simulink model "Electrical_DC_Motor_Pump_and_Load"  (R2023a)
settings: Solver=VariableStepAuto  StartTime=0.0  StopTime=10.0  RelTol=1e-3
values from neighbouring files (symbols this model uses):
  K_q = 1    [Electrical_DC_Motor_Pump_and_Load_EQN.m]    (also in Electrical_DC_Motor_Pump_and_Load_SLX_m.m; Electrical_DC_Motor_and_Pump_EQN.m; Electrical_DC_Motor_and_Pump_SLX_m.m)
  K_t = 1    [Electrical_DC_Motor_Pump_and_Load_EQN.m]    (also in Electrical_DC_Motor_Pump_and_Load_SLX_m.m; Electrical_DC_Motor_and_Pump_EQN.m; Electrical_DC_Motor_and_Pump_SLX_m.m)
undefined symbols (not defined in the file or in its folder): eTr, rGi
libraries: fl_lib x14

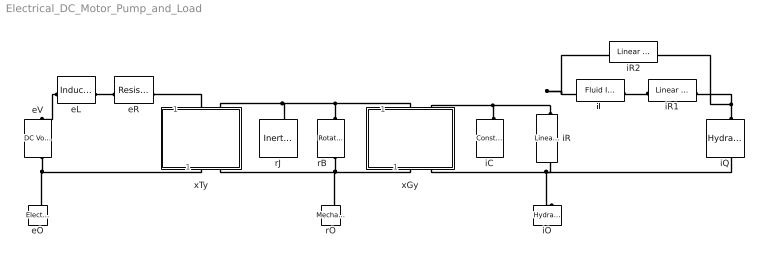
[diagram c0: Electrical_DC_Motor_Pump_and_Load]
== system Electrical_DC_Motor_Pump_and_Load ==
  eL : fl_lib/Electrical/Electrical Elements/Inductor  l=1e-6 H  r=0 Ohm  g=1e-9 1/Ohm  i_specify=off  i_priority=None  i=0 A  i_nominal_specify=off  i_nominal_unit=A  i_nominal_value=1  v_specify=off  v_priority=None  v=0 V  v_nominal_specify=off  v_nominal_unit=V  v_nominal_value=1  i_L_specify=off  i_L_priority=High  i_L=0 A  i_L_nominal_specify=off  i_L_nominal_unit=A  i_L_nominal_value=1
  eO : fl_lib/Electrical/Electrical Elements/Electrical Reference
  eR : fl_lib/Electrical/Electrical Elements/Resistor  R=1 Ohm  i_specify=off  i_priority=None  i=0 A  i_nominal_specify=off  i_nominal_unit=A  i_nominal_value=1  v_specify=off  v_priority=None  v=0 V  v_nominal_specify=off  v_nominal_unit=V  v_nominal_value=1
  eV : fl_lib/Electrical/Electrical Sources/DC Voltage Source  v0=1 V
  iC : fl_lib/Hydraulic/Hydraulic Elements/Constant Volume Hydraulic Chamber  ch_sp=foundation.enum.chamberGeometry.volume  wall_type=foundation.enum.chamber_spec.rigid  ch_volume=1e-4 m^3  d_in=1e-2 m  length=1 m  pr_r_coef=1.2e-12 m/Pa  time_const=0.01 s  k_sh=1.4  pressure_specify=off  pressure_priority=High  pressure=0 Pa  pressure_nominal_specify=off  pressure_nominal_unit=Pa  pressure_nominal_value=1  diameter_incr_specify=off  diameter_incr_priority=High  diameter_incr=0 m  diameter_incr_nominal_specify=off  diameter_incr_nominal_unit=m  diameter_incr_nominal_value=1  flow_rate_specify=off  flow_rate_priority=None  flow_rate=1e-3 m^3/s  flow_rate_nominal_specify=off  flow_rate_nominal_unit=m^3/s  flow_rate_nominal_value=1
  iL : fl_lib/Hydraulic/Hydraulic Elements/Fluid Inertia  area=0.8e-4 m^2  length=1 m  q_specify=off  q_priority=High  q=1e-3 m^3/s  q_nominal_specify=off  q_nominal_unit=m^3/s  q_nominal_value=1  p_specify=off  p_priority=None  p=0 Pa  p_nominal_specify=off  p_nominal_unit=Pa  p_nominal_value=1
  iO : fl_lib/Hydraulic/Hydraulic Elements/Hydraulic Reference
  iQ : fl_lib/Hydraulic/Hydraulic Sources/Hydraulic Constant Flow Rate Source  commanded_flow_rate=0.001 m^3/s
  iR : fl_lib/Hydraulic/Hydraulic Elements/Linear Hydraulic Resistance  resistance=10e9 Pa*s/m^3  q_specify=off  q_priority=None  q=1e-3 m^3/s  q_nominal_specify=off  q_nominal_unit=m^3/s  q_nominal_value=1  p_specify=off  p_priority=None  p=0 Pa  p_nominal_specify=off  p_nominal_unit=Pa  p_nominal_value=1
  iR1 : fl_lib/Hydraulic/Hydraulic Elements/Linear Hydraulic Resistance  resistance=10e9 Pa*s/m^3  q_specify=off  q_priority=None  q=1e-3 m^3/s  q_nominal_specify=off  q_nominal_unit=m^3/s  q_nominal_value=1  p_specify=off  p_priority=None  p=0 Pa  p_nominal_specify=off  p_nominal_unit=Pa  p_nominal_value=1
  iR2 : fl_lib/Hydraulic/Hydraulic Elements/Linear Hydraulic Resistance  resistance=10e9 Pa*s/m^3  q_specify=off  q_priority=None  q=1e-3 m^3/s  q_nominal_specify=off  q_nominal_unit=m^3/s  q_nominal_value=1  p_specify=off  p_priority=None  p=0 Pa  p_nominal_specify=off  p_nominal_unit=Pa  p_nominal_value=1
  rB : fl_lib/Mechanical/Rotational Elements/Rotational Damper  D=0.001 N*m*s/rad  w_specify=off  w_priority=None  w=0 rad/s  w_nominal_specify=off  w_nominal_unit=rad/s  w_nominal_value=1  t_specify=off  t_priority=None  t=0 N*m  t_nominal_specify=off  t_nominal_unit=N*m  t_nominal_value=1
  rJ : fl_lib/Mechanical/Rotational Elements/Inertia  inertia=0.01 kg*m^2  num_ports=foundation.enum.numPorts2.one  w_specify=off  w_priority=High  w=0 rad/s  w_nominal_specify=off  w_nominal_unit=rad/s  w_nominal_value=1  t_specify=off  t_priority=None  t=0 N*m  t_nominal_specify=off  t_nominal_unit=N*m  t_nominal_value=1
  rO : fl_lib/Mechanical/Rotational Elements/Mechanical Rotational Reference
  xGy : Subsystem  mask{Gyrator_type=rGi, G_type=F2=K*E1, xGy=K_q}
      mask prompts: Gyrator_type "Type of Gytator"; G_type "Type of relation"; xGy "Name of parameter K"
  xTy : Subsystem  mask{Transformer_type=eTr, T_type=F2=K*F1, xTy=K_t}
      mask prompts: Transformer_type "Type of Transformer"; T_type "Type of relation"; xTy "Name of parameter K"
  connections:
  eV/RConn1 -- xTy/RConn1 -- eO/LConn1
  eL/LConn1 -- eV/LConn1
  eR/LConn1 -- eL/RConn1
  xTy/LConn1 -- eR/RConn1
  rB/LConn1 -- xGy/LConn1 -- xTy/LConn2 -- rJ/LConn1
  rB/RConn1 -- rO/LConn1 -- xGy/RConn1 -- xTy/RConn2
  xGy/RConn2 -- iR/RConn1 -- iQ/RConn1 -- iO/LConn1
  iR/LConn1 -- iR2/LConn1 -- iL/LConn1 -- xGy/LConn2 -- iC/LConn1
  iR1/LConn1 -- iL/RConn1
  iQ/LConn1 -- iR2/RConn1 -- iR1/RConn1

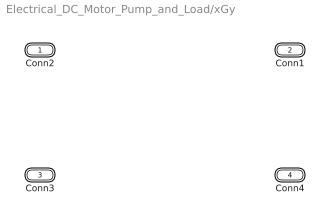
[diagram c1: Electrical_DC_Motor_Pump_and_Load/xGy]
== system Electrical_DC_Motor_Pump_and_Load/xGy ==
  Conn2 : PMIOPort  Side=Left
  Conn1 : PMIOPort  Port=2  Side=Left
  Conn3 : PMIOPort  Port=3  Side=Right
  Conn4 : PMIOPort  Port=4  Side=Right

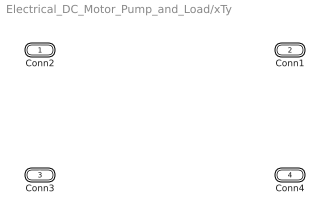
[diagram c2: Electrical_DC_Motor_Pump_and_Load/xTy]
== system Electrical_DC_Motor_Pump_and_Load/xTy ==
  Conn2 : PMIOPort  Side=Left
  Conn1 : PMIOPort  Port=2  Side=Left
  Conn3 : PMIOPort  Port=3  Side=Right
  Conn4 : PMIOPort  Port=4  Side=Right
